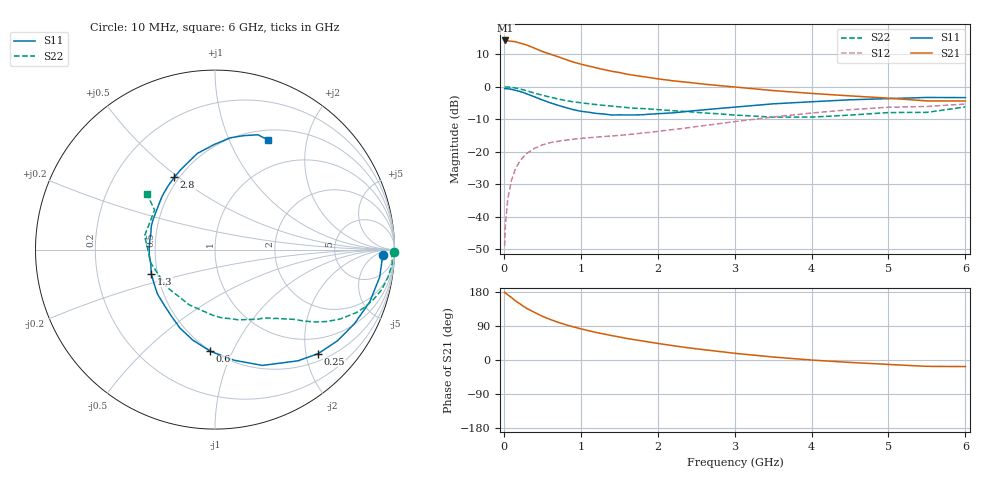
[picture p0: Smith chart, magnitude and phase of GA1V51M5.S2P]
! Infineon Technologies  Discrete & RF Semiconductors
! BF775
! Si NPN RF Bipolar Junction Transistor in SOT23
! VCE = 1.5 V  IC = 1.5 mA
! Common Emitter S-Parameters:  May  1996
# GHz  S  MA  R  50
!  f  S11  S21  S12  S22
! GHz  MAG  ANG  MAG  ANG  MAG  ANG  MAG  ANG
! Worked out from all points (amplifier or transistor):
!   36 points, 10 MHz to 6 GHz, reference 50 ohm
!   highest |S21| = 14.2 dB at 20 MHz (marker M1)
!   |S21| within 3 dB of that: start of sweep to 459.9 MHz
!   unconditionally stable (mu >= 1): 1.241 GHz to end of sweep
!   at 250 MHz: K = 0.25, MSG = 17.4 dB, |S12| = -21.7 dB
!   at 1.4 GHz: K = 1.09, MAG = 8.1 dB, |S12| = -15.2 dB
!   at 6 GHz: K = 1.05, MAG = -0.9 dB, |S12| = -5.3 dB
!   S11 on the Smith chart (normalised r, x): 10 MHz: 24, -12; 250 MHz: 0.65, -2.24; 600 MHz: 0.49, -0.82; 1.3 GHz: 0.46, -0.14; 2.8 GHz: 0.47, +0.48; 6 GHz: 0.62, +1.40
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0.01  0.9349 -1.9  5.055 178.8  0.0035 87.7  0.9972 -0.9
0.02  0.9326 -3.7  5.153 176.8  0.0073 91.8  0.9854 -1.8
0.05  0.9304 -9.5  5.098 172.2  0.0183 83.3  0.9907 -4.6
0.1  0.91 -18.7  5.003 164.8  0.0366 78.3  0.9761 -9.1
0.15  0.8796 -28.0  4.933 156.2  0.0537 72.8  0.9545 -13.6
0.25  0.816 -45.3  4.552 142.5  0.082 63.6  0.8963 -20.8
0.3  0.773 -53.3  4.374 135.9  0.0943 59.7  0.8625 -24.0
0.4  0.6974 -67.7  3.914 125.6  0.1125 52.8  0.7964 -29.1
0.5  0.6256 -80.2  3.48 115.4  0.1267 47.5  0.7395 -32.8
0.6  0.5666 -92.7  3.179 107.2  0.1372 43.6  0.6912 -35.7
0.7  0.5187 -103.9  2.905 99.8  0.1442 41.0  0.6488 -38.0
0.8  0.4788 -114.1  2.634 93.3  0.1498 38.7  0.6123 -40.0
0.9  0.4437 -123.1  2.402 87.6  0.1553 37.4  0.5851 -41.6
1.1  0.405 -142.4  2.082 77.5  0.1638 35.4  0.5467 -44.9
1.3  0.3795 -159.3  1.833 68.6  0.1712 34.9  0.5154 -48.0
1.6  0.367 178.1  1.559 56.8  0.1825 36.1  0.4773 -53.0
2.2  0.3954 144.3  1.231 37.8  0.2188 38.8  0.4267 -66.0
2.8  0.4622 119.4  1.04 22.5  0.2696 38.4  0.3821 -84.3
3.5  0.5445 100.5  0.872 7.9  0.341 33.7  0.3396 -114.9
4.5  0.6285 82.3  0.722 -6.4  0.4425 21.9  0.3652 -168.1
5.5  0.6831 69.5  0.604 -16.8  0.4962 6.6  0.4023 146.7
6  0.6788 64.3  0.602 -17.3  0.5407 2.4  0.4885 140.9
